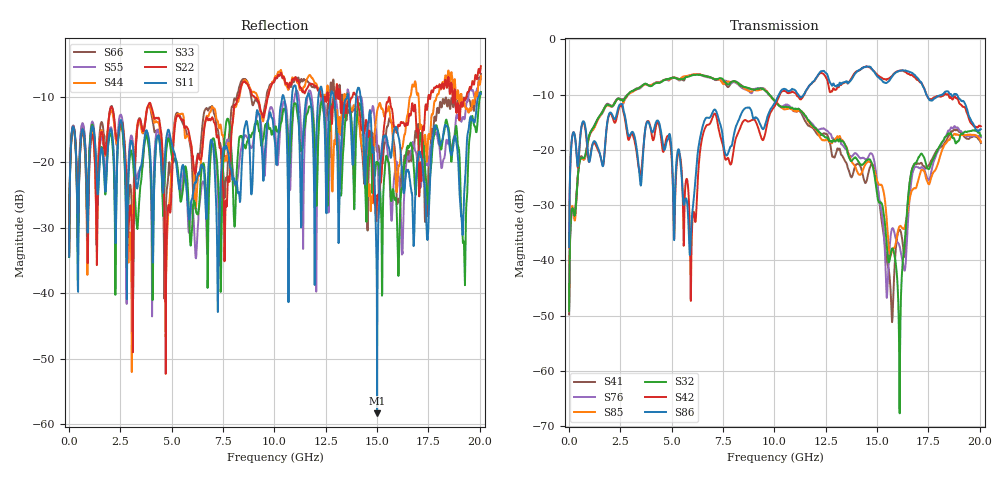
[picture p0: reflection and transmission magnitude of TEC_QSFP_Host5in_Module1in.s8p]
!!  This file represents Tyco Electronics parts only.  Due to internal design and materials, it should not  !!
!!  be used for products manufactured by companies other than Tyco Electronics.  !!
!! FILE NAME: TEC_QSFP_Host5in_Module1in.s8p
!! PART DESCRIPTION: Tyco Electronics QSFP P/N 1761987-9
!! PCB DESCRIPTION: Host Board FR4 with 5 inch microstrip, Module Board FR4 with 1.5 inch microstrip
!! FILE DESCRIPTION: 8 Port, S-Parameter, Measured Channel
!! FILE REVISION: Revision 2, 3/12/2008
!! FILE FREQUENCY RANGE: DC to 20.05 GHz in 12.50 MHz frequency steps
!! PORT DEFINITIONS:
!! Port  1  ----->  Host	Pin 24, RX4-	Module  <-----  Port  2
!! Port  3  ----->  Host	Pin 25, RX4+	Module  <-----  Port  4
!! Port  5  ----->  Host	Pin 33, TX3+	Module  <-----  Port  6
!! Port  7  ----->  Host	Pin 34, TX3-	Module  <-----  Port  8
# HZ S MA R 50.00
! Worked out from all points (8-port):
!   1604 points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, 12.5 MHz to 20.05 GHz, reference 50 ohm
!   strongest paths, dB at 12.5 MHz, 5.025 GHz, 10.04 GHz, 15.05 GHz, 20.05 GHz:
!     S86: -37.6, -21.9, -11.4, -6.8, -16.2
!     S42: -37.6, -23.1, -11.9, -6.5, -15.7
!     S32: -49.1, -7.0, -11.3, -29.1, -17.5
!     S85: -48.3, -7.0, -11.2, -26.0, -18.5
!     S76: -48.7, -7.0, -11.1, -27.3, -17.7
!     S41: -49.8, -6.9, -11.2, -27.3, -18.7
!   lowest |S11| = -58.3 dB at 15 GHz (marker M1), VSWR 1.00, Z = 50 + j0.121 ohm
!   |S11| at or under -10 dB: start of sweep to 10.39 GHz; 12.9 GHz to 13.55 GHz (652 MHz wide, 4.93 % of centre); 14.2 GHz to 19.94 GHz (5.742 GHz wide, 33.6 % of centre)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
